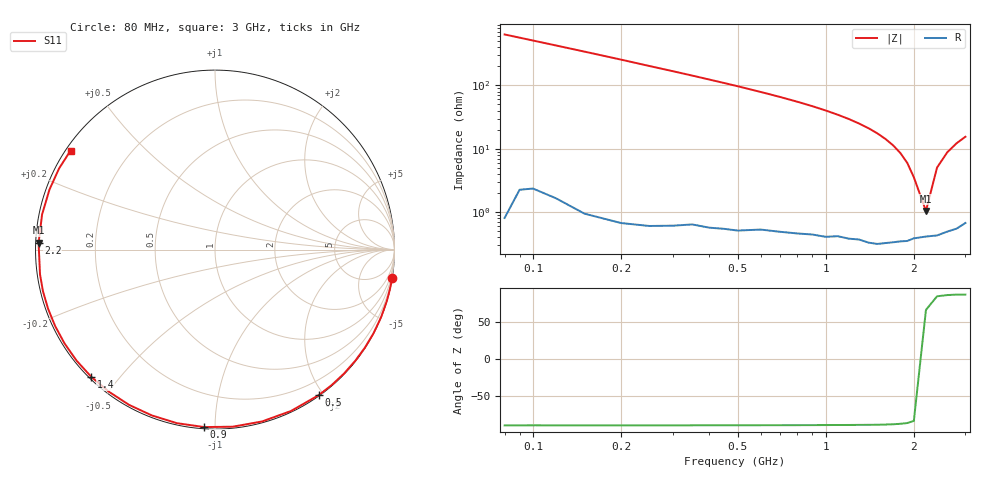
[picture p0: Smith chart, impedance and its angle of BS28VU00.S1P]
! SIEMENS Small Signal Semiconductors
! BB640
! Si Tuning Diode in SOD323
! VR = 28 V
! S-Parameters:  July  1993
# GHz  S  MA  R  50
!  f  S11
! GHz  MAG  ANG
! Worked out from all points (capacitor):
!   33 points, 80 MHz to 3 GHz, reference 50 ohm
!   read as one part to ground: C = 3.12 pF near 80 MHz
!   lowest |Z| = 1.05 ohm at 2.2 GHz (marker M1)
!   series resonance near 2.157 GHz, so ESL is about 1.7 nH
!   S11 on the Smith chart (normalised r, x): 80 MHz: 0, -13; 500 MHz: 0.01, -1.94; 900 MHz: 0.01, -0.94; 1.4 GHz: 0.01, -0.42; 2.2 GHz: 0.01, +0.02; 3 GHz: 0.01, +0.31
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0.08  0.9998 -9.0
0.15  0.9992 -16.7
0.2  0.999 -22.2
0.25  0.9986 -27.8
0.3  0.998 -33.2
0.35  0.9972 -38.6
0.45  0.9962 -49.3
0.5  0.9957 -54.5
0.6  0.9939 -64.8
0.7  0.9928 -74.7
0.8  0.9917 -84.3
0.9  0.9906 -93.5
1  0.9901 -102.4
1.1  0.9887 -110.9
1.2  0.9887 -119.0
1.3  0.9882 -126.8
1.4  0.9888 -134.2
1.5  0.9888 -141.3
1.6  0.988 -148.1
1.7  0.9873 -154.5
1.8  0.9866 -160.6
1.9  0.9862 -166.4
2  0.9847 -171.9
2.2  0.9836 177.8
2.4  0.9831 168.5
2.6  0.981 160.1
2.8  0.9794 152.5
3  0.9756 145.6
